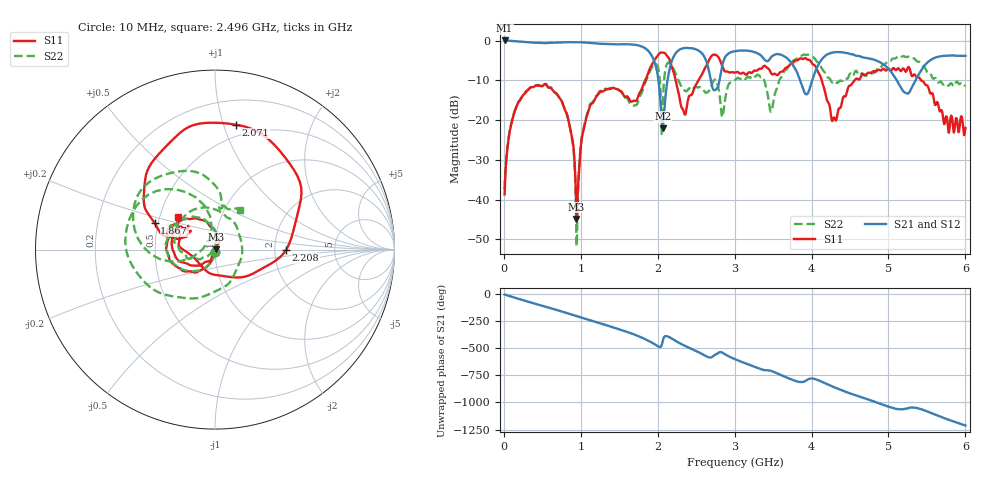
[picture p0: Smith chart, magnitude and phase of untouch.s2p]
!  15/09/2025  16:02:58
! Ref Plane: 0.000 mm
# MHZ S MA R  50
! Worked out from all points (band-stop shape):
!   1001 points, 10 MHz to 6 GHz, reference 50 ohm
!   highest |S21| = 0.02 dB at 10 MHz (marker M1); lowest = -22.1 dB at 2.065 GHz (marker M2)
!   |S21| within 3 dB of the highest: start of sweep to 1.894 GHz; 2.242 GHz to 2.563 GHz (321 MHz wide, 13.4 % of centre)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
!   lowest |S11| = -44.9 dB at 944.4 MHz (marker M3), VSWR 1.01, Z = 50.5 + j0.231 ohm
!   |S11| at or under -10 dB: start of sweep to 1.838 GHz; 4.132 GHz to 4.561 GHz (428.1 MHz wide, 9.85 % of centre); 5.425 GHz to end of sweep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
!   |S22| runs from -51.7 to -3.5 dB; largest |S21 - S12| = 0.012
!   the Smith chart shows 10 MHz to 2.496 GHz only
!   S11 on the Smith chart (normalised r, x): 10 MHz: 1.00, -0.02; 1.867 GHz: 0.48, +0.16; 2.071 GHz: 0.40, +1.10; 2.208 GHz: 2.31, -0.01; 2.496 GHz: 0.62, +0.25
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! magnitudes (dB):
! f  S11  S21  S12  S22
! 10 MHz  -38.7  0.0  0.0  -37.3
! 165.7 MHz  -16.6  -0.2  -0.3  -16.5
! 537.1 MHz  -10.9  -0.7  -0.7  -10.7
! 824.6 MHz  -18.8  -0.4  -0.5  -18.9
! 944.4 MHz  -44.9  -0.4  -0.5  -51.7
! 1.01 GHz  -25.0  -0.5  -0.5  -24.7
! 1.232 GHz  -13.4  -0.8  -0.8  -13.1
! 1.867 GHz  -8.7  -2.4  -2.4  -9.3
! 2.011 GHz  -3.5  -10.1  -10.2  -7.2
! 2.065 GHz  -3.0  -22.1  -22.1  -17.9
! 2.071 GHz  -3.0  -21.2  -21.2  -14.2
! 2.208 GHz  -8.0  -4.0  -4.1  -7.3
! 2.34 GHz  -18.0  -1.9  -1.9  -12.4
! 2.496 GHz  -11.2  -2.2  -2.3  -11.7
! 2.741 GHz  -3.6  -12.5  -12.5  -9.8
! 2.843 GHz  -6.7  -6.0  -6.0  -19.2
! 3.005 GHz  -8.1  -2.7  -2.7  -9.9
! 3.478 GHz  -8.3  -4.1  -4.1  -17.8
! 4.005 GHz  -5.7  -10.1  -10.1  -4.1
! 4.293 GHz  -19.3  -3.0  -3.0  -10.2
! 5.006 GHz  -7.0  -7.3  -7.3  -5.1
! 6 GHz  -22.0  -3.9  -3.9  -11.2
